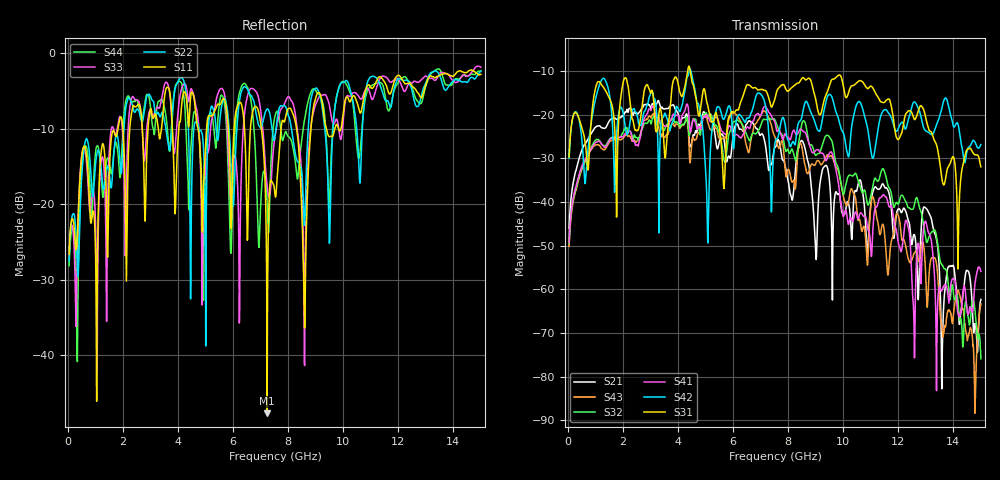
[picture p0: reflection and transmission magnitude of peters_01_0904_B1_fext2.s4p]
# MHZ S RI R 50.00
! FREQ  S11  S12  S13  S14
!  S21  S22  S23  S24
!  S31  S32  S33  S34
!  S41  S42  S43  S44
!  REAL  IMAG  REAL  IMAG  REAL  IMAG  REAL  IMAG
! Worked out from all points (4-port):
!   1496 points, 50 MHz to 15 GHz, reference 50 ohm
!   strongest paths, dB at 50 MHz, 3.79 GHz, 7.53 GHz, 11.27 GHz, 15 GHz:
!     S31: -29.7, -13.6, -16.2, -16.1, -31.9
!     S42: -30.0, -21.9, -26.3, -23.1, -26.8
!     S41: -49.3, -20.6, -21.9, -40.1, -55.9
!     S32: -49.5, -21.1, -21.3, -35.2, -75.9
!     S43: -50.2, -22.2, -25.2, -45.0, -63.3
!     S21: -46.0, -17.8, -27.5, -37.1, -62.3
!   lowest |S11| = -47.7 dB at 7.24 GHz (marker M1), VSWR 1.01, Z = 50.3 - j0.323 ohm
!   |S11| at or under -10 dB: start of sweep to 1.824 GHz; 7.031 GHz to 7.744 GHz (713.2 MHz wide, 9.65 % of centre); 8.308 GHz to 8.83 GHz (521.6 MHz wide, 6.09 % of centre)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
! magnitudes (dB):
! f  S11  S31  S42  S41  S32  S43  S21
! 50 MHz  -26.6  -29.7  -30.0  -49.3  -49.5  -50.2  -46.0
! 3.62 GHz  -4.5  -24.2  -21.2  -22.6  -22.2  -24.6  -18.6
! 4.47 GHz  -5.6  -11.0  -10.0  -23.9  -23.4  -29.1  -27.2
! 5.08 GHz  -8.6  -17.8  -48.7  -20.6  -20.6  -21.7  -20.9
! 7.24 GHz  -47.7  -15.1  -20.2  -18.7  -21.1  -20.0  -30.1
! 12.56 GHz  -4.5  -20.8  -17.2  -65.3  -41.3  -52.0  -47.5
! 15 GHz  -2.8  -31.9  -26.8  -55.9  -75.9  -63.3  -62.3
